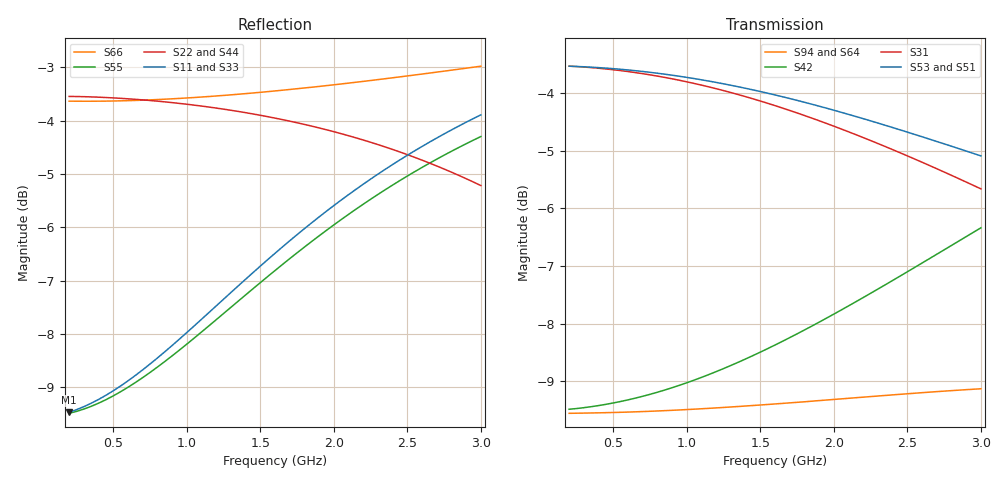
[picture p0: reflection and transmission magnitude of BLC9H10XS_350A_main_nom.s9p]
! Touchstone file from project LM8HV_ModelValidation_separatedPorts_AW_1
! Exported from HFSS 2017.0.0
! Variables:
!  AirBoxH = 25000um
!  AirBoxL = 30000um
!  AirBoxW = 55000um
!  BW_Xoffset = 0mm
!  BW_Yoffset = 0mm
!  BW_Zoffset = 0mm
!  Lb1_LH = 0.865mm
!  Lb1_SP = 1.03mm
!  Lg3_LH = 1.115mm
!  Lg3_SP = 3.76mm
!  PCB_H = 760um
!  X0_Lb1 = 1.03mm
!  X0_Lg3 = 0mm
!  X1_Lb1 = 0.80031mm
!  X1_Lg3 = 0.79712mm
!  X2_Lb1 = 0.71688mm
!  X2_Lg3 = 1.0528mm
!  X3_Lb1 = 0.5768mm
!  X3_Lg3 = 1.34608mm
!  X4_Lb1 = 0.4841mm
!  X4_Lg3 = 1.77096mm
!  X5_Lb1 = 0mm
!  X5_Lg3 = 3.76mm
!  Z0_Lb1 = 0.7114mm
!  Z0_Lg3 = 0.7114mm
!  Z1_Lb1 = 0.83905mm
!  Z1_Lg3 = 1.0481mm
!  Z2_Lb1 = 0.867595mm
!  Z2_Lg3 = 1.111655mm
!  Z3_Lb1 = 0.858945mm
!  Z3_Lg3 = 1.12169mm
!  Z4_Lb1 = 0.82175mm
!  Z4_Lg3 = 1.035835mm
!  Z5_Lb1 = 0.05mm
!  Z5_Lg3 = 0.05mm
# GHZ S MA R 50.000000
! Terminal data exported
! Port[1] = 2EDD
! Port[2] = 2EGD
! Port[3] = 4
! Port[4] = 2
! Port[5] = BB_Drain_T1
! Port[6] = BB_Gate1_T1
! Port[7] = BB_Gate2_T1
! Port[8] = BB_Gate3_T1
! Port[9] = BB_Gate4_T1
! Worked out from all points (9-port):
!   57 points, 200 MHz to 3 GHz, reference per port
!   strongest paths, dB at 200 MHz, 900 MHz, 1.6 GHz, 2.3 GHz, 3 GHz:
!     S53: -3.5, -3.7, -4.0, -4.5, -5.1
!     S51: -3.5, -3.7, -4.0, -4.5, -5.0
!     S31: -3.5, -3.8, -4.2, -4.9, -5.7
!     S42: -9.5, -9.1, -8.4, -7.4, -6.3
!     S94: -9.6, -9.5, -9.4, -9.3, -9.1
!     S64: -9.6, -9.5, -9.4, -9.3, -9.1
!   lowest |S11| = -9.5 dB at 200 MHz (marker M1), VSWR 2.01
!   |S11| at or under -10 dB: nowhere
